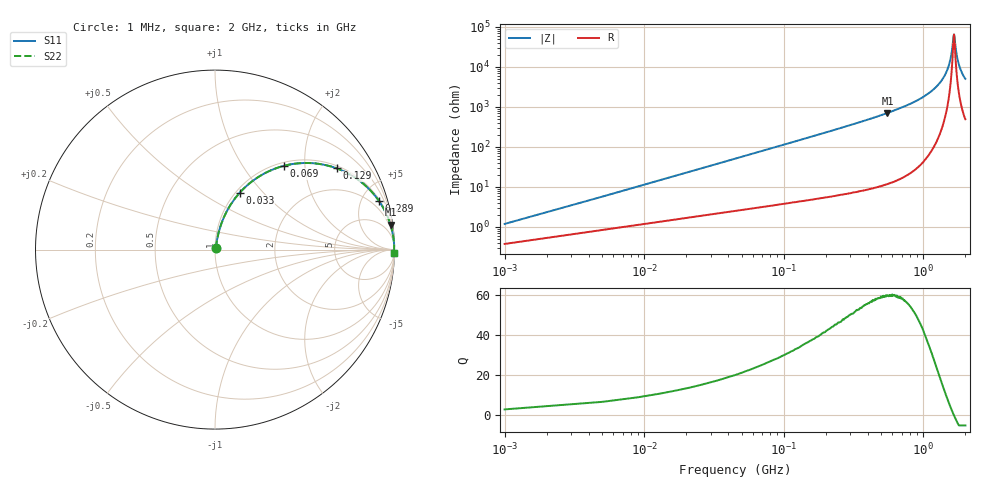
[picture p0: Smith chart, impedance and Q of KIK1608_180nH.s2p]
!version-2
!date-01.2022
!Series
# MHz S RI R 50
!Freq ReS11 ImS11 ReS21 ImS21 ReS12 ImS12 ReS22 ImS22
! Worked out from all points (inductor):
!   501 points, 1 MHz to 2 GHz, reference 50 ohm
!   read as one part in series: L = 180 nH near 9 MHz
!   highest Q = 59.7 at 553 MHz (marker M1), where L = 202 nH
!   self-resonance near 1.657 GHz
!   S11 on the Smith chart (normalised r, x): 1 MHz: 1.01, +0.02; 33 MHz: 1.04, +0.75; 69 MHz: 1.06, +1.56; 129 MHz: 1.09, +2.94; 289 MHz: 1.14, +6.74; 2 GHz: open
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1  0.00387 0.0112  0.9961 -0.0112  0.9961 -0.0112  0.00387 0.0112
13  0.0337 0.1402  0.9663 -0.1402  0.9663 -0.1402  0.0337 0.1402
21  0.0678 0.2177  0.9322 -0.2177  0.9322 -0.2177  0.0678 0.2177
33  0.1365 0.3156  0.8635 -0.3156  0.8635 -0.3156  0.1365 0.3156
69  0.3842 0.4668  0.6158 -0.4668  0.6158 -0.4668  0.3842 0.4668
129  0.6783 0.4526  0.3217 -0.4526  0.3217 -0.4526  0.6783 0.4526
193  0.8246 0.3684  0.1754 -0.3684  0.1754 -0.3684  0.8246 0.3684
289  0.9145 0.2696  0.0854 -0.2696  0.0854 -0.2696  0.9145 0.2696
337  0.9366 0.2344  0.0634 -0.2344  0.0634 -0.2344  0.9366 0.2344
553  0.978 0.1387  0.022 -0.1387  0.022 -0.1387  0.978 0.1387
669  0.9861 0.109  0.0139 -0.109  0.0139 -0.109  0.9861 0.109
1003  0.9956 0.0554  0.00442 -0.0554  0.00442 -0.0554  0.9956 0.0554
1337  0.9981 0.0229  0.00185 -0.0229  0.00185 -0.0229  0.9981 0.0229
1450  0.9984 0.0143  0.00159 -0.0143  0.00159 -0.0143  0.9984 0.0143
1530  0.9985 0.00854  0.00152 -0.00854  0.00152 -0.00854  0.9985 0.00854
1590  0.9985 0.00446  0.00151 -0.00446  0.00151 -0.00446  0.9985 0.00446
1645  0.9985 0.000796  0.00154 -0.000796  0.00154 -0.000796  0.9985 0.000796
1670  0.9984 -0.000736  0.00156 0.000736  0.00156 0.000736  0.9984 -0.000736
1720  0.9984 -0.00398  0.00163 0.00398  0.00163 0.00398  0.9984 -0.00398
1780  0.9983 -0.00761  0.00174 0.00761  0.00174 0.00761  0.9983 -0.00761
1880  0.998 -0.0134  0.00198 0.0134  0.00198 0.0134  0.998 -0.0134
2000  0.9977 -0.0198  0.00234 0.0198  0.00234 0.0198  0.9977 -0.0198
